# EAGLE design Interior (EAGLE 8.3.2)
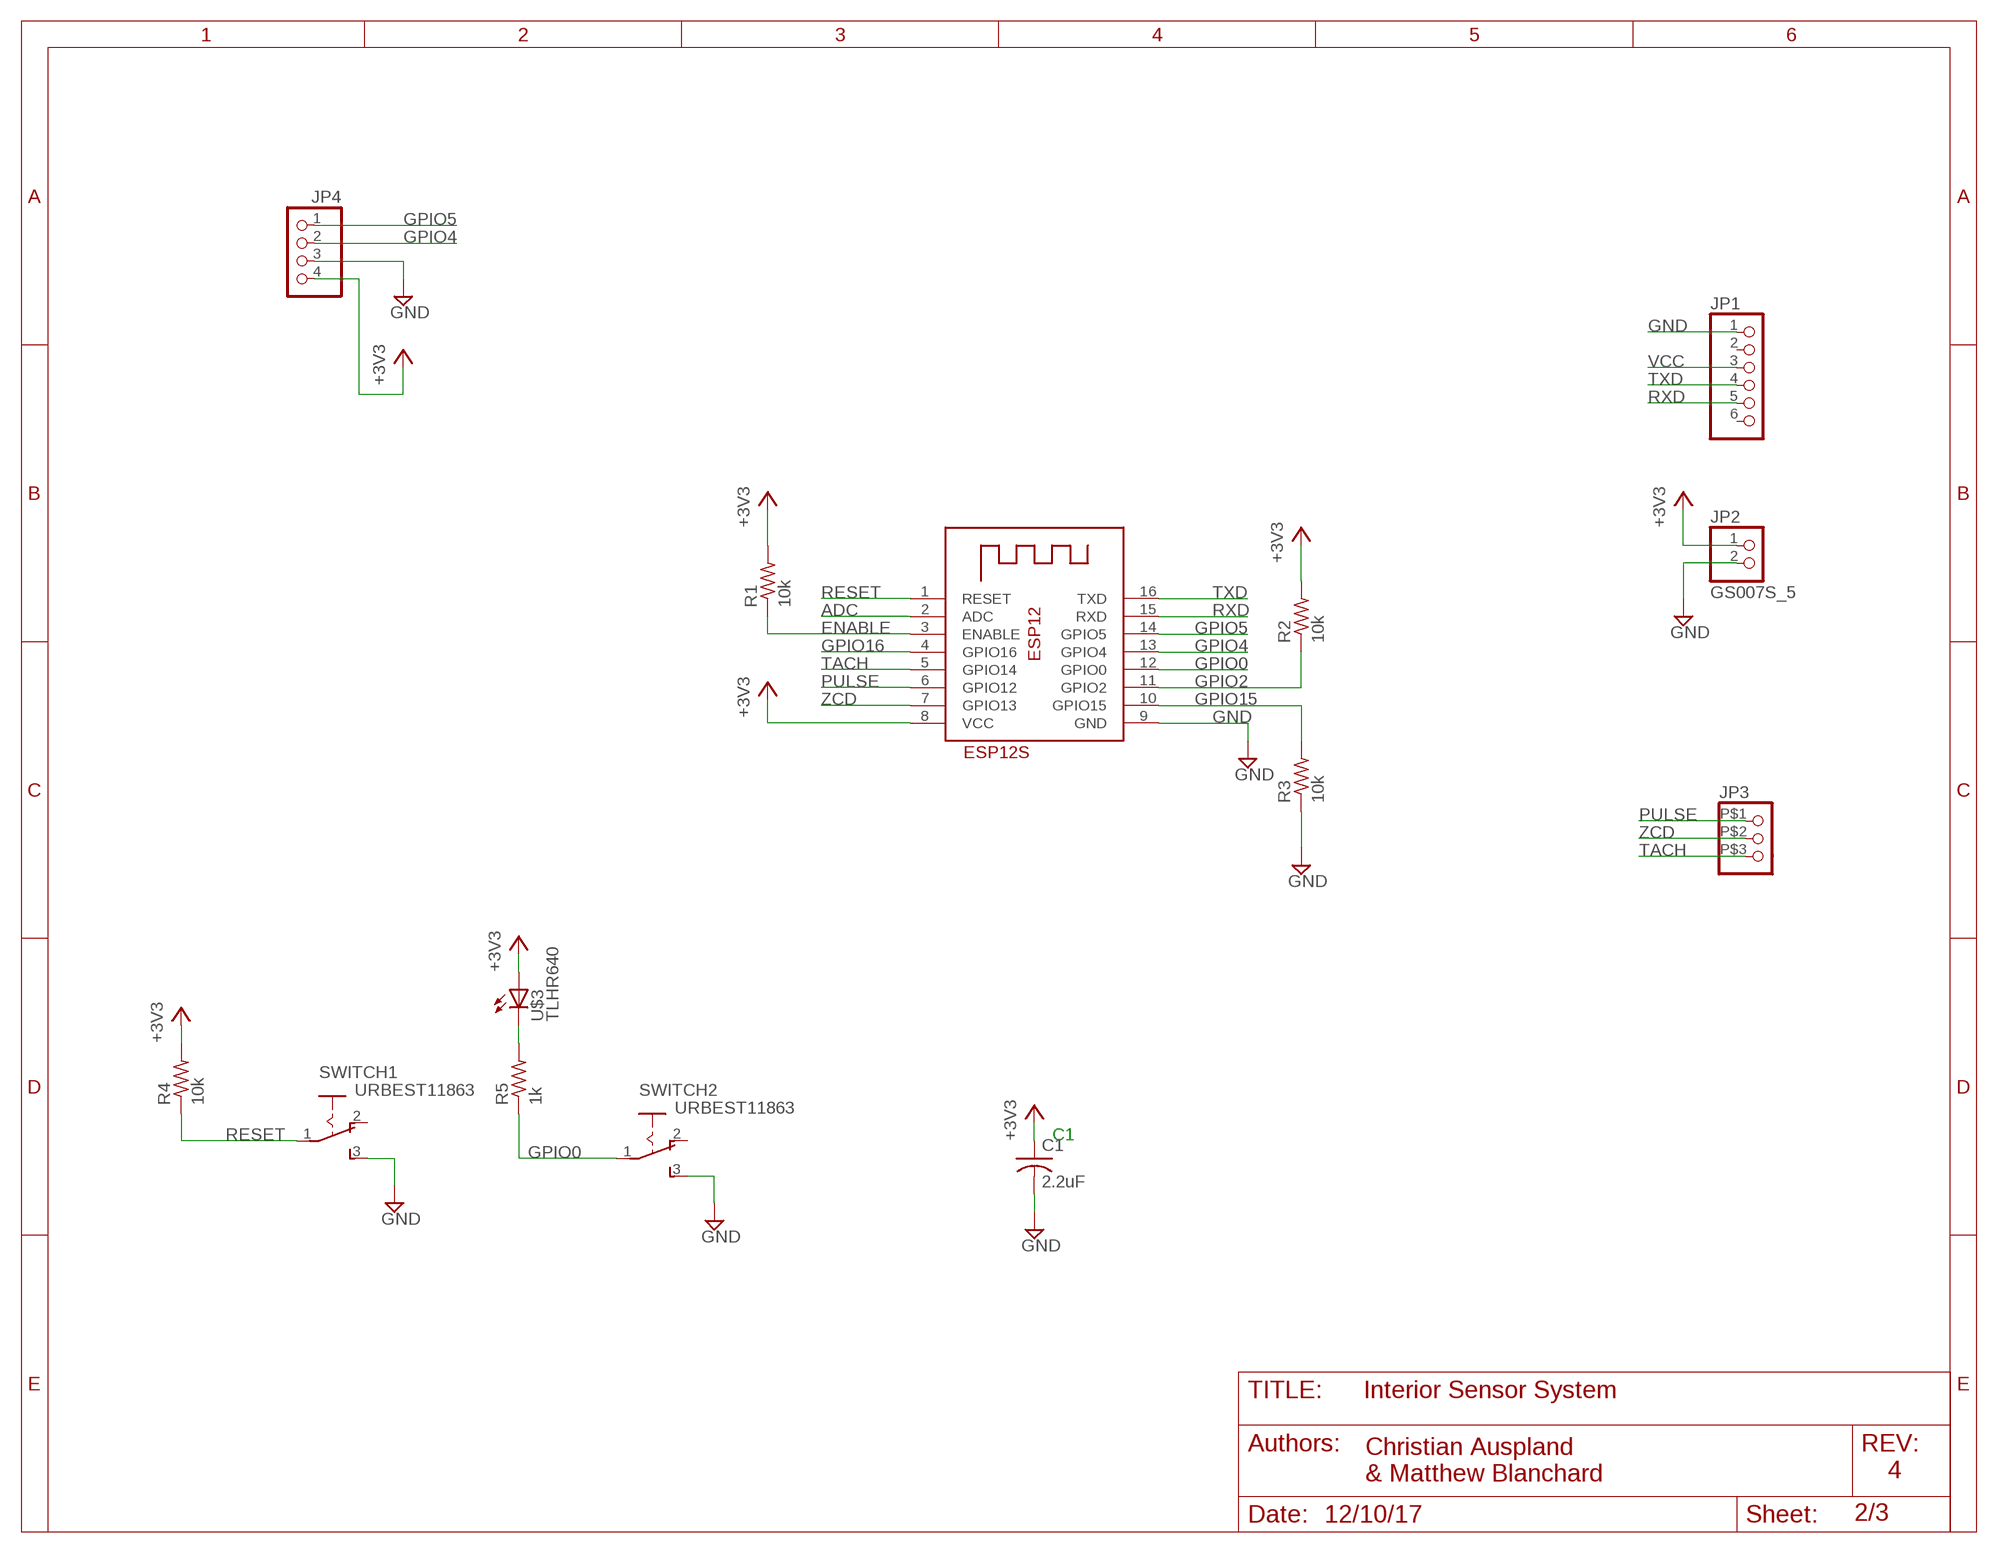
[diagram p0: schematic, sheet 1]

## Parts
C1  2.2uF  CAP  [MYCAP]
ESP12S  MYESP12S  [MYESP12S]
JP1  PINHD-1X6  [1X06]
JP2  GS007S_5  [GS007S_5]
JP3  GSOO19_2.54_3P  [GSO19_2.54_3P]
JP4  PINHD-1X4  [1X04]
R1  10k  R10K  [R10K]
R2  10k  R10K  [R10K]
R3  10k  R10K  [R10K]
R4  10k  R10K  [R10K]
R5  1k  R10K  [R10K]
SWITCH1  URBEST11863  [URBEST11863]
SWITCH2  URBEST11863  [URBEST11863]
U$3  TLHR640  [TLHR640]

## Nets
+3V3: C1.P ESP12S.8(VCC) JP2.1 JP4.4 R1.2 R2.2 R4.2 U$3.A
ADC: ESP12S.2(ADC)
ENABLE: ESP12S.3(ENABLE) R1.1
GND: C1.M ESP12S.9(GND) JP1.1 JP2.2 JP4.3 R3.1 SWITCH1.3(GND) SWITCH2.3(GND)
GPIO0: ESP12S.12(GPIO0) R5.1 SWITCH2.1(RESET)
GPIO2: ESP12S.11(GPIO2) R2.1
GPIO4: ESP12S.13(GPIO4) JP4.2
GPIO5: ESP12S.14(GPIO5) JP4.1
GPIO15: ESP12S.10(GPIO15) R3.2
GPIO16: ESP12S.4(GPIO16)
N$4: R5.2 U$3.C
PULSE: ESP12S.6(GPIO12) JP3.P$1
RESET: ESP12S.1(RESET) R4.1 SWITCH1.1(RESET)
RXD: ESP12S.15(RXD) JP1.5
TACH: ESP12S.5(GPIO14) JP3.P$3
TXD: ESP12S.16(TXD) JP1.4
VCC: JP1.3
ZCD: ESP12S.7(GPIO13) JP3.P$2
Unconnected: JP1.2 JP1.6 SWITCH1.2(VCC) SWITCH2.2(VCC)

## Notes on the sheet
- C1
- Interior Sensor System
- 4
- Christian Auspland 
  & Matthew Blanchard
- 12/10/17 | 2/3

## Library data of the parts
C1 = MyLibrary:CAP
ESP12S = MyLibrary:MYESP12S
JP1 = adafruit:PINHD-1X6: PIN HEADER
JP2 = MyLibrary:GS007S_5
JP3 = MyLibrary:GSOO19_2.54_3P
JP4 = pinhead:PINHD-1X4: PIN HEADER
R1-R5 = MyLibrary:R10K
SWITCH1 SWITCH2 = MyLibrary:URBEST11863
U$3 = MyLibrary:TLHR640

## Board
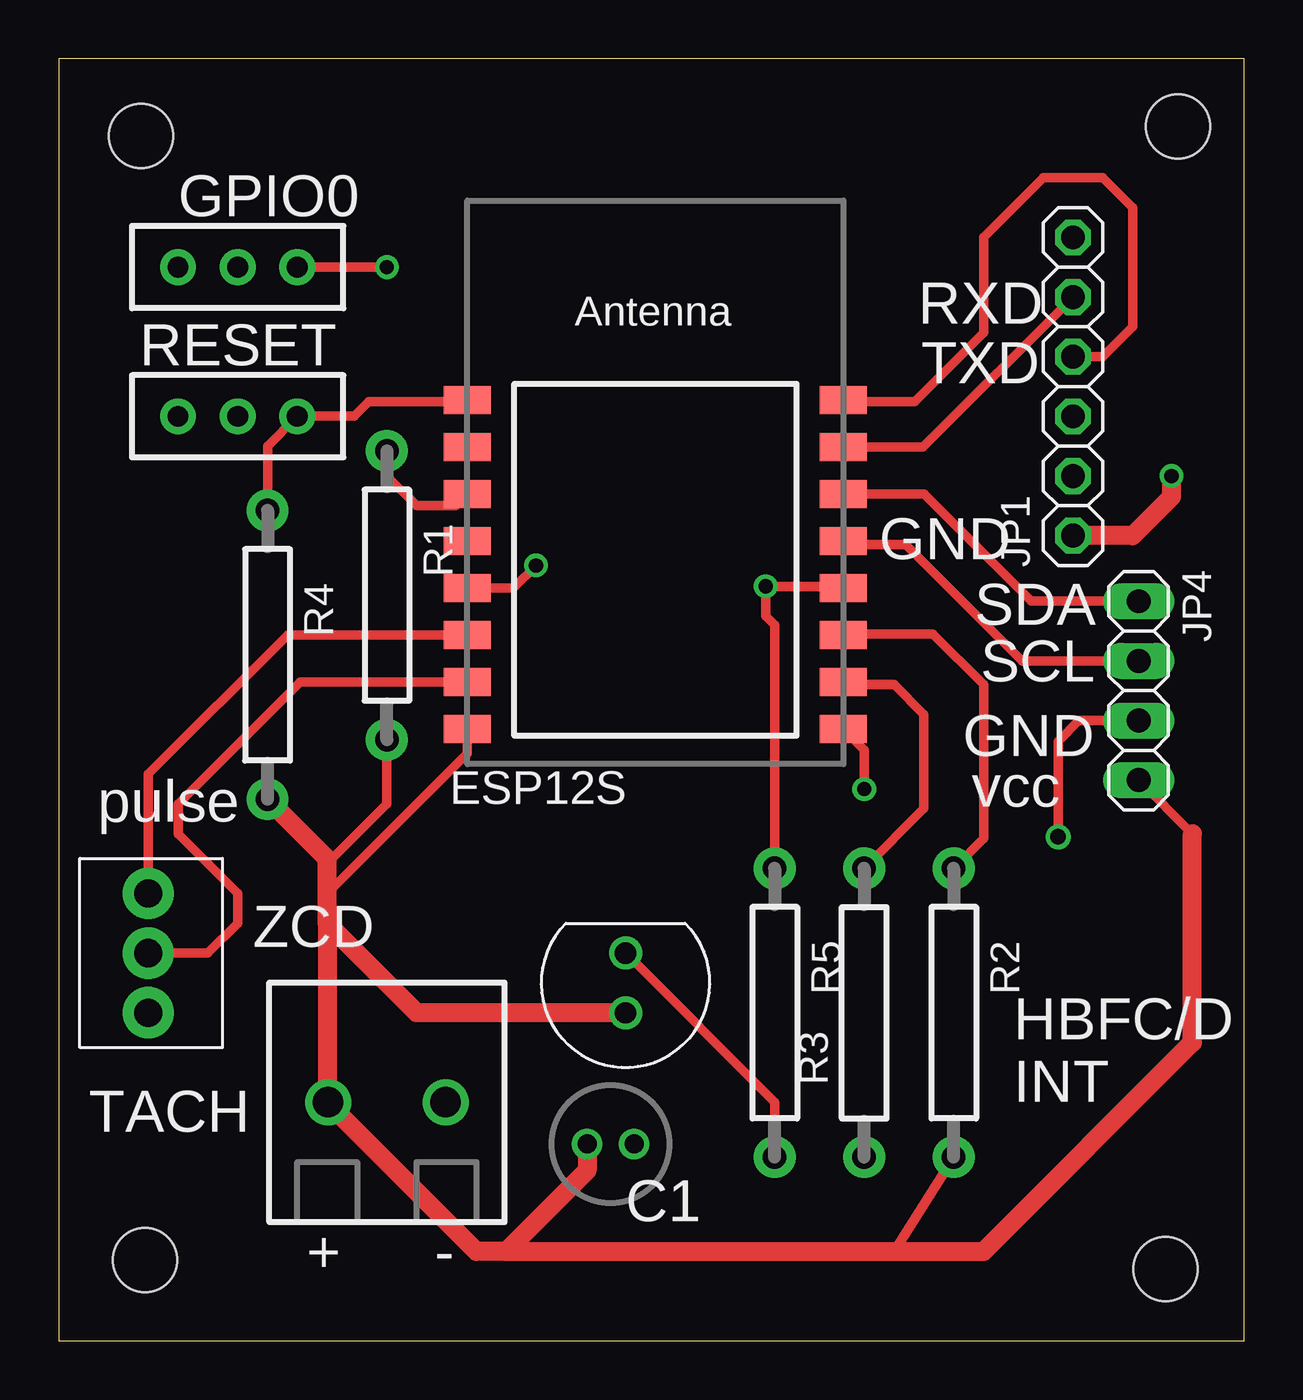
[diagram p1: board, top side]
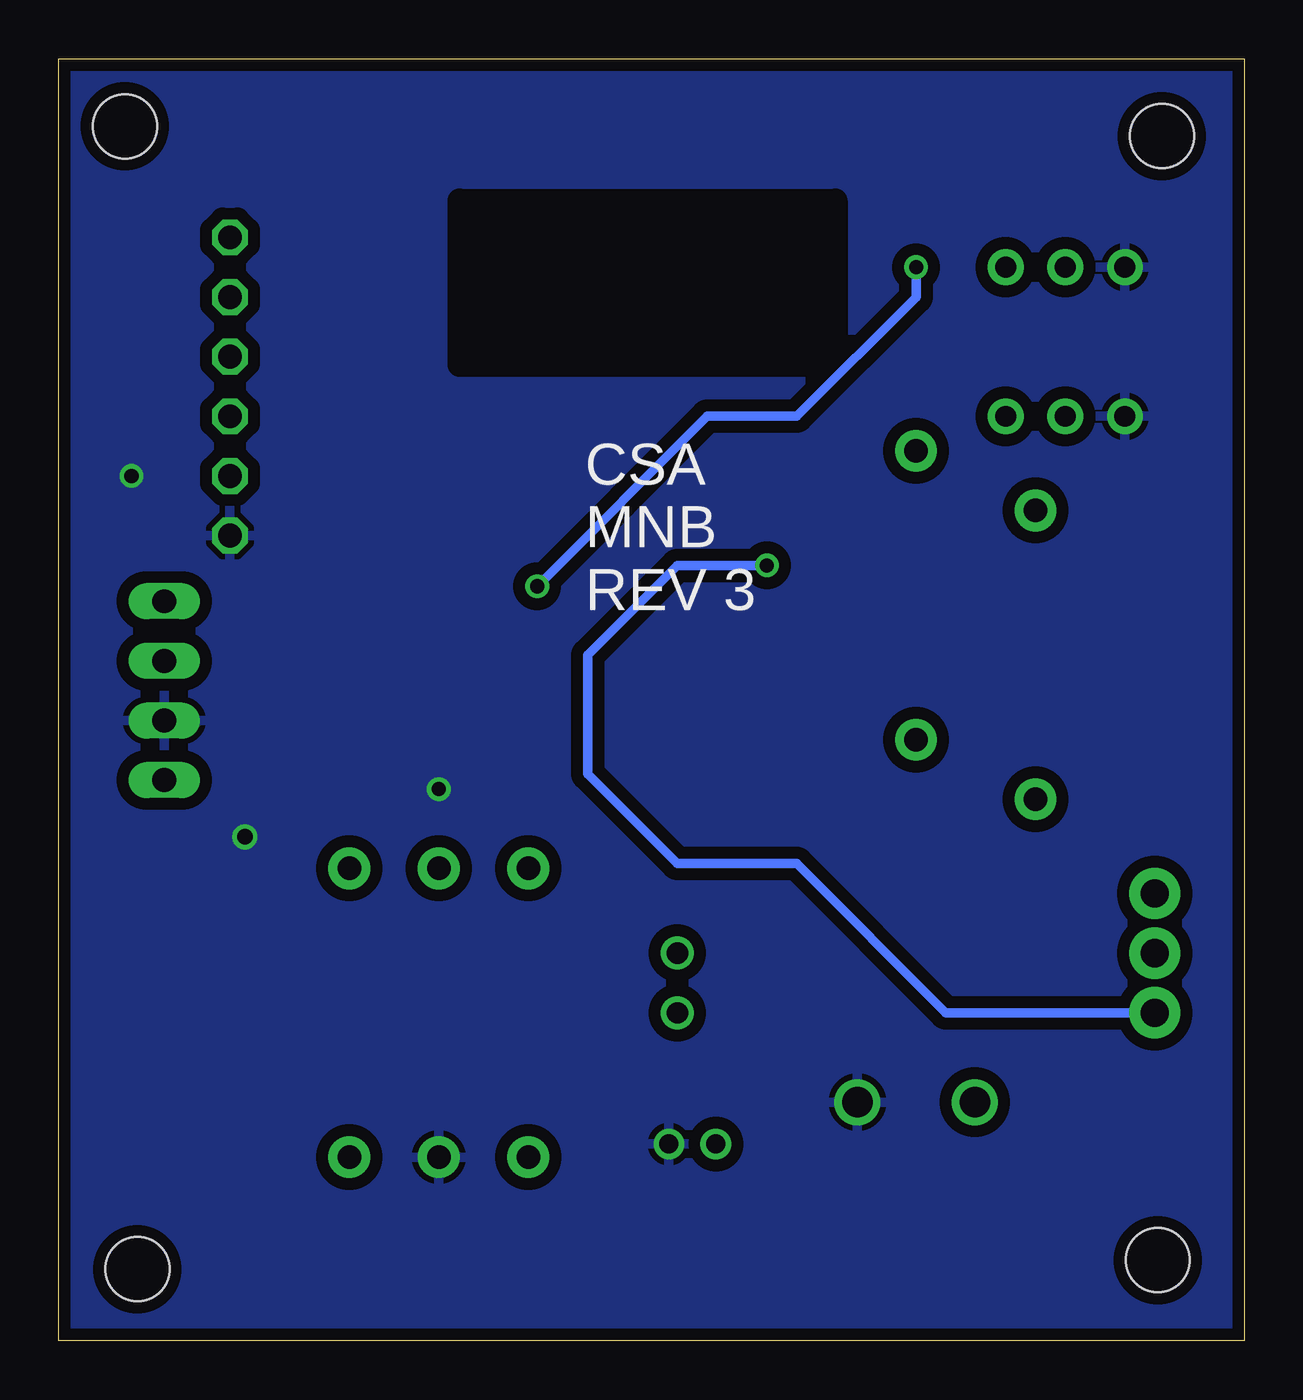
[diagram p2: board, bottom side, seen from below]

Size 50.47 x 54.6 mm. Coordinates in mm from the lower left corner, seen from the top.
Outline: 0,0 50.47,0 50.47,54.6 0,54.6 0,0
Copper layers (1*16): Top 0.035mm / dielectric 1.5mm / Bottom 0.035mm
Design rules "default *": minimum track width 10mil, minimum drill 15mil, track to track 10mil, track to pad 10mil, pad to pad 10mil, via to via 10mil, smd to smd 6mil, copper to edge 15mil, drill to drill 15mil, minimum pad ring 10mil, minimum via ring 8mil, stop-mask expansion 4mil, vias tented up to drill 0mil, thermal gap 10mil
Holes 2.73 mm at 3.68,3.43 47.12,3.05 47.66,51.72 3.51,51.31

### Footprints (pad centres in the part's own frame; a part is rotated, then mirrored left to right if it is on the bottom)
MYCAP = drill 0.8: M 1,0; P -1,0
MYESP12S = smd 2 x 1.2: 1 -8,4.5; 2 -8,2.5; 3 -8,0.5; 4 -8,-1.5; 5 -8,-3.5; 6 -8,-5.5; 7 -8,-7.5; 8 -8,-9.5; 9 8,-9.5; 10 8,-7.5; 11 8,-5.5; 12 8,-3.5; 13 8,-1.5; 14 8,0.5; 15 8,2.5; 16 8,4.5
1X06 = drill 1.016 octagon: 1 -6.35,0; 2 -3.81,0; 3 -1.27,0; 4 1.27,0; 5 3.81,0; 6 6.35,0
GS007S_5 = drill 1.3: 1 -2.5,0; 2 2.5,0
GSO19_2.54_3P = drill 1.2 pad 2.184: P$1 -2.54,2.54; P$2 0,2.54; P$3 2.54,2.54
1X04 = drill 1.016 long: 1 -3.81,0; 2 -1.27,0; 3 1.27,0; 4 3.81,0
R10K = drill 1 pad 1.778: 1 -6.15,0; 2 6.15,0
URBEST11863 = drill 0.889 pad 1.524: 1 -2.54,0; 2 0,0; 3 2.54,0
TLHR640 = drill 0.9: A -1.27,0; C 1.27,0

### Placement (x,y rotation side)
C1  23.5,8.38 0 top
ESP12S  25.4,35.56 0 top
JP1  43.18,40.64 90 top
JP2  13.97,10.16 0 top
JP3  1.27,16.51 270 top
JP4  45.97,27.69 270 top
R1  13.97,31.75 270 top
R2  38.1,13.97 270 top
R3  34.29,13.97 90 top
R4  8.89,29.21 270 top
R5  30.48,13.97 270 top
SWITCH1  7.62,39.37 180 top
SWITCH2  7.62,45.72 180 top
U$3  24.13,15.24 90 top

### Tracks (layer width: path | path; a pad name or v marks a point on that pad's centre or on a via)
+3V3
  Top 0.406: 35.56,3.81 R2.2 | 48.26,21.59 JP4.4 | 11.43,20.32 13.97,22.86 R1.2 | 11.43,19.05 17.4,25.02 ESP12S.8
  Top 0.813: 48.26,21.59 48.26,12.7 39.37,3.81 35.56,3.81 19.05,3.81 | 11.43,17.78 11.43,19.05 11.43,20.32 11.43,20.52 R4.2 | 11.43,17.78 11.43,10.2 JP2.1 11.47,10.12 17.78,3.81 19.05,3.81 | U$3.A 15.24,13.97 11.43,17.78 | C1.P 22.5,7.26 19.05,3.81
ENABLE
  Top 0.406: R1.1 13.97,36.83 15.24,35.56 16.9,35.56 ESP12S.3
GND  (via drill 0.6, 0.65)
  Top 0.406: v34.29,23.49 34.29,25.17 ESP12S.9 | v42.55,21.46 42.55,25.53 43.43,26.42 JP4.3
  Top 0.813: v47.37,36.83 47.37,35.94 45.72,34.29 JP1.1
  pour Bottom (isolate 0.508): 0,0 0,54.61 50.8,54.61 50.8,0
GPIO0  (via drill 0.6)
  Top 0.406: ESP12S.12 33.33,32.13 v30.1,32.13 30.1,30.86 30.48,30.48 R5.1 | SWITCH2.1 v13.97,45.72
  Bottom 0.406: v30.1,32.13 22.86,39.37 19.05,39.37 13.97,44.45 v13.97,45.72
GPIO2
  Top 0.406: ESP12S.11 33.44,30.1 37.21,30.1 39.37,27.94 39.37,21.39 R2.1
GPIO4
  Top 0.406: 35.94,33.91 35.56,33.91 | 35.56,33.91 33.55,33.91 ESP12S.13 | 35.56,33.91 36.07,33.91 41.02,28.96 JP4.2
GPIO5
  Top 0.406: JP4.1 41.4,31.5 36.84,36.06 ESP12S.14
GPIO15
  Top 0.406: ESP12S.10 33.52,27.94 35.56,27.94 36.83,26.67 36.83,22.66 R3.2
N$4
  Top 0.406: R5.2 30.48,10.16 U$3.C
PULSE
  Top 0.406: 17.18,29.84 ESP12S.6 9.74,30.06 3.81,24.13 JP3.P$1
RESET
  Top 0.406: ESP12S.1 17.34,40 13.21,40 12.57,39.37 SWITCH1.1 8.89,38.1 R4.1
RXD
  Top 0.406: JP1.5 36.79,38.06 ESP12S.15
TACH  (via drill 0.6)
  Top 0.406: v20.32,33.02 19.36,32.06 ESP12S.5
  Bottom 0.406: v20.32,33.02 24.13,33.02 27.94,29.21 27.94,24.13 24.13,20.32 19.05,20.32 12.7,13.97 JP3.P$3
TXD
  Top 0.406: JP1.4 44.45,41.91 45.72,43.18 45.72,48.26 44.45,49.53 41.91,49.53 39.37,46.99 39.37,42.93 36.45,40 33.46,40 ESP12S.16
ZCD
  Top 0.406: 17.28,27.94 ESP12S.7 10.28,28.06 5.08,22.86 5.08,21.59 7.62,19.05 7.62,17.78 6.35,16.51 JP3.P$2

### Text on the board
tPlace: GPIO0 | RXD | RESET | TXD | GND | SDA | SCL | GND | vcc | pulse | ZCD | HBFC/D / INT | TACH | C1 | + | -
bPlace: CSA / MNB / REV 3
